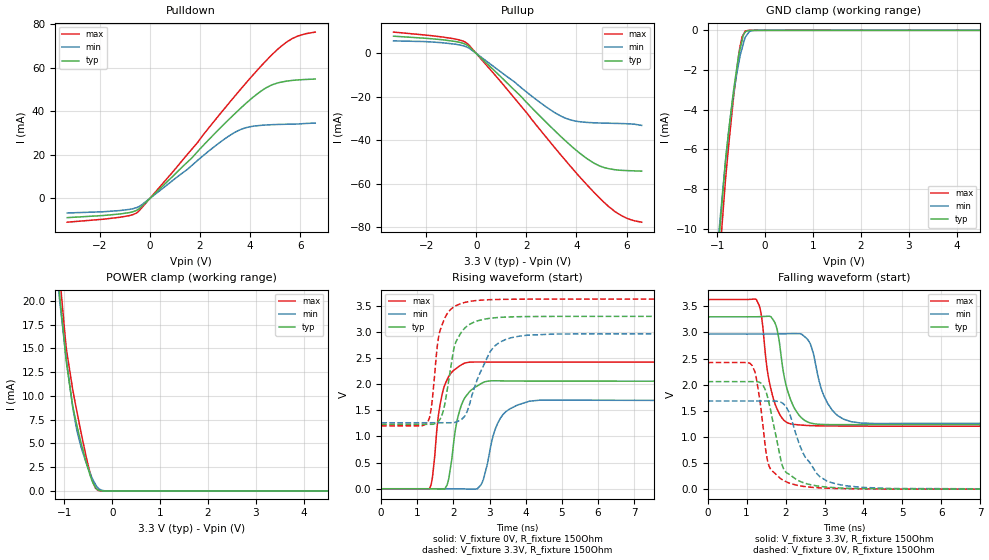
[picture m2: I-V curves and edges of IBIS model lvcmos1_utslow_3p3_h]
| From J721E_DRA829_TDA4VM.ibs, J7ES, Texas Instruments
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|   utslow_3p3_h
[Model]   lvcmos1_utslow_3p3_h
Model_type   I/O
Polarity   Non-Inverting
Enable   Active-High
Vinl = 0
Vinh = 0.8
Vmeas = 1.65
Vref = 3.3
Cref = 2pF
Rref = 100000
|   typ   min   max
C_comp   1.414pF   1.380pF   1.447pF
[Voltage Range]   3.3   2.97   3.63
[Temperature Range]   27   150   -40
[Pullup Reference]   3.3   2.97   3.63
[Pulldown Reference]   0   0   0
[Power Clamp Reference]   3.3   2.97   3.63
[GND Clamp Reference]   0   0   0
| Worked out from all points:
|   slope of the pulldown table from 0 to 0.495 V, typ, clamps not added: 90 ohm
|   slope of the pullup table from 0 to 0.495 V, typ, clamps not added: 91.4 ohm
|   GND clamp passes 1 mA (typ) near -0.53 V on its own axis
|   POWER clamp passes 1 mA (typ) near -0.42 V on its own axis
|   falling waveform, V_fixture 3.3V, R_fixture 150Ohm: 20-80 % time 341ps typ, 413ps min, 293ps max; typ from 3.3 V to 1.23 V
|   rising waveform, V_fixture 0V, R_fixture 150Ohm: 20-80 % time 327ps typ, 411ps min, 277ps max; typ from 0 V to 2.06 V
|   rising waveform, V_fixture 3.3V, R_fixture 150Ohm: 20-80 % time 361ps typ, 581ps min, 278ps max; typ from 1.23 V to 3.3 V
|   falling waveform, V_fixture 0V, R_fixture 150Ohm: 20-80 % time 361ps typ, 620ps min, 268ps max; typ from 2.06 V to 0 V
[Pulldown]
|   Voltage   I(typ)   I(min)   I(max)
-3.3V     -8.812mA   -6.674mA   -10.9mA
-1.191V   -7.125mA   -5.554mA   -8.631mA
-518.1mV  -5.375mA   -4.179mA   -6.575mA
1.67V     18.52mA    15.08mA    22.53mA
2.779V    31.96mA    25.57mA    38.45mA
3.561V    40.74mA    31.3mA     49.27mA
4.026V    45.55mA    32.96mA    55.48mA
4.66V     50.89mA    33.72mA    63.46mA
5.105V    53.01mA    33.95mA    68.49mA
5.442V    53.8mA     34.04mA    71.64mA
5.917V    54.39mA    34.17mA    74.56mA
6.6V      54.79mA    34.58mA    76.34mA
[GND Clamp]
|   Voltage   I(typ)   I(min)   I(max)
-3.3V     -115mA     -82.92mA   -162mA
-1.023V   -12.29mA   -11.74mA   -13.78mA
-825mV    -6.567mA   -6.574mA   -7.512mA
-696.3mV  -3.81mA    -3.895mA   -4.302mA
-656.7mV  -3.034mA   -3.217mA   -3.362mA
-557.7mV  -1.363mA   -1.768mA   -1.395mA
-478.5mV  -504.3uA   -900.3uA   -329.3uA
-448.8mV  -224.5uA   -642.1uA   -196.6uA
-409.2mV  -83.52uA   -334uA     -32.8uA
-320.1mV  -4.75uA    -57.38uA   -1.332uA
-132mV    -59.88nA   -1.582uA   -94.69nA
6.6V      0A         0A         0A
[Pullup]
|   Voltage   I(typ)   I(min)   I(max)
-3.3V     7.968mA    5.806mA    9.861mA
-1.33V    6.298mA    4.923mA    7.574mA
-686.4mV  5.198mA    3.984mA    6.273mA
-359.7mV  3.766mA    2.847mA    4.622mA
996.6mV   -10.95mA   -8.669mA   -13.26mA
3.105V    -35.3mA    -27.06mA   -43.04mA
3.749V    -42.25mA   -30.58mA   -51.87mA
4.422V    -48.52mA   -31.79mA   -60.63mA
4.976V    -52.08mA   -32.07mA   -67.27mA
5.531V    -53.59mA   -32.23mA   -72.85mA
6.026V    -54mA      -32.41mA   -76.06mA
6.6V      -54.25mA   -33.16mA   -77.79mA
[POWER Clamp]
|   Voltage   I(typ)   I(min)   I(max)
-3.3V     170.4mA    144.6mA    202.9mA
-1.132V   22.5mA     21.65mA    24.88mA
-1.092V   20.32mA    19.77mA    22.37mA
-953.7mV  13.38mA    13.61mA    14.77mA
-825mV    8.921mA    8.795mA    10.65mA
-745.8mV  7.051mA    6.572mA    8.54mA
-627mV    4.601mA    4.228mA    5.562mA
-478.5mV  1.925mA    2.067mA    2.209mA
-409.2mV  924.1uA    1.225mA    995.8uA
-300.3mV  125uA      342.8uA    57.84uA
-23.1mV   2.435nA    849.9nA    21nA
6.6V      0A         0A         0A
[Ramp]
R_load = 150
|   typ   min   max
dV/dt_r   1.2349/3.25887e-10   1.01256/4.11146e-10   1.45469/2.77266e-10
dV/dt_f   1.23995/3.38282e-10   1.02414/4.08252e-10   1.45527/2.92519e-10
[Falling Waveform]
V_fixture = 3.3V
V_fixture_min = 2.97V
V_fixture_max = 3.63V
R_fixture = 150Ohm
C_fixture = 0F
|   Time   V(typ)   V(min)   V(max)
0s        3.3V       2.97V      3.63V
1.255ns   3.3V       2.97V      3.625V
1.37ns    3.303V     2.97V      3.375V
1.54ns    3.31V      2.97V      2.241V
1.725ns   3.19V      2.97V      1.645V
2.105ns   1.766V     2.977V     1.256V
2.57ns    1.285V     2.863V     1.219V
3.075ns   1.237V     1.65V      1.211V
3.68ns    1.235V     1.293V     1.207V
10ns      1.233V     1.263V     1.204V
[Rising Waveform]
V_fixture = 0V
V_fixture_min = 0V
V_fixture_max = 0V
R_fixture = 150Ohm
C_fixture = 0F
|   Time   V(typ)   V(min)   V(max)
0s        121.5uV    304.9uV    70.76uV
1.335ns   11.99uV    256.4uV    -2.266mV
1.715ns   -7.451mV   164.7uV    1.887V
1.85ns    135.7mV    150uV      2.124V
2.075ns   1.216V     -1.474mV   2.302V
2.305ns   1.73V      -3.849mV   2.403V
2.79ns    2.023V     113.3mV    2.425V
3.37ns    2.064V     1.419V     2.424V
4.1ns     2.06V      1.675V     2.424V
10ns      2.058V     1.688V     2.425V
[Rising Waveform]
V_fixture = 3.3V
V_fixture_min = 2.97V
V_fixture_max = 3.63V
R_fixture = 150Ohm
C_fixture = 0F
|   Time   V(typ)   V(min)   V(max)
0s        1.233V     1.263V     1.204V
1.285ns   1.233V     1.263V     1.275V
1.39ns    1.233V     1.263V     1.562V
1.63ns    1.331V     1.263V     3.03V
1.755ns   1.599V     1.263V     3.256V
2.02ns    2.706V     1.266V     3.484V
2.195ns   2.97V      1.314V     3.541V
3.015ns   3.262V     2.622V     3.619V
3.595ns   3.289V     2.889V     3.626V
10ns      3.3V       2.97V      3.63V
[Falling Waveform]
|Gnd
V_fixture = 0V
V_fixture_min = 0V
V_fixture_max = 0V
R_fixture = 150Ohm
C_fixture = 0F
|   Time   V(typ)   V(min)   V(max)
0s        2.058V     1.688V     2.425V
1.135ns   2.058V     1.688V     2.376V
1.255ns   2.058V     1.687V     2.108V
1.57ns    1.668V     1.687V     458.5mV
1.91ns    472.4mV    1.653V     184.7mV
2.155ns   252.5mV    1.333V     102.4mV
2.44ns    128.8mV    705.6mV    55.2mV
2.79ns    64.3mV     310.6mV    28.77mV
3.31ns    26.36mV    98.02mV    13.21mV
10ns      121.5uV    305.5uV    70.78uV
